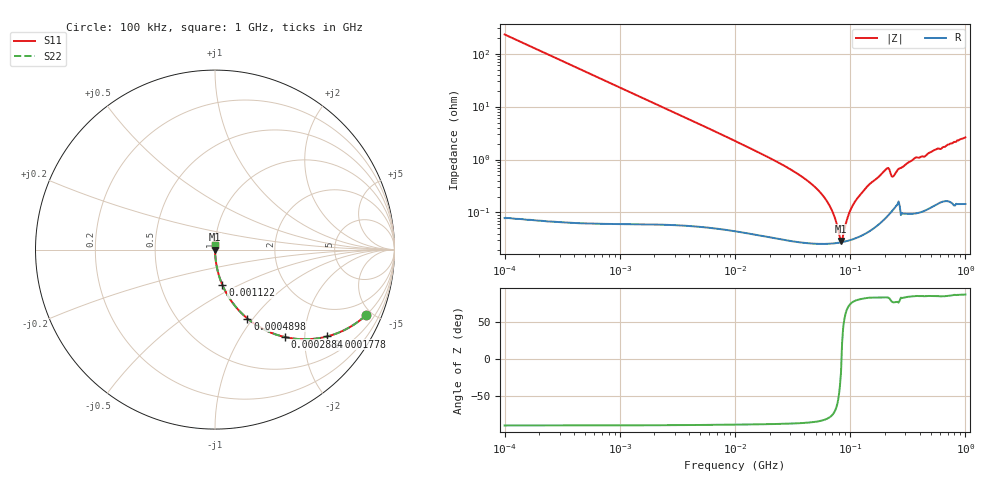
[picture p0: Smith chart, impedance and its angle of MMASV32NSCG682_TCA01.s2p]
! MMASV32NSCG682_TCA01  S-PARAMETER MODEL  ( Standard Model )
! Model Generated by TAIYO YUDEN Corporation (https://www.yuden.co.jp/en/)
! Version 1.0
! TAIYO YUDEN Control No. 250312
! Copyright(c) 2025 TAIYO YUDEN CO.,LTD. All Rights Reserved.
! Product Description (link to TY-COMPAS)
! https://ds.yuden.co.jp/TYCOMPAS/or/detail?pn=MMASV32NSCG682JTCA01&u=M
! Products Name : Multilayer Ceramic Capacitors
! Characteristics :
!  Capacitance : 6800 [pF] , Rated Voltage : 1000 [V] , TCC : CG / C0G
!  Case Size : 3.2 x 2.5 / 0.126 x 0.098 [mm/inch] , Thickness : 1.9 / 0.075 [mm/inch]
!  (Conditions: Temperature = 25 [degC] , DC Bias Voltage = 0 [V])
! External Node Assignments :
!  1  o---| |---o  2
! GND o---------o GND
! Frequency Range : 0.1MHz  -  1000MHz  [ 401 STEP ]
# MHZ S RI R 50
! Freq[MHz].  S11 Real  S11 Imag  S21 Real  S21 Imag  S12 Real  S12 Imag  S22 Real  S22 Imag
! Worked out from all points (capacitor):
!   401 points, 100 kHz to 1 GHz, reference 50 ohm
!   read as one part in series: C = 6.92 nF near 104.7 kHz
!   lowest |Z| = 28.9 mohm at 83.18 MHz (marker M1)
!   series resonance near 84.05 MHz, so ESL is about 520 pH
!   S11 on the Smith chart (normalised r, x): 100 kHz: 1.00, -4.60; 177.8 kHz: 1.00, -2.59; 288.4 kHz: 1.00, -1.60; 489.8 kHz: 1.00, -0.94; 1.122 MHz: 1.00, -0.41; 1 GHz: 1.00, +0.05
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0.1  0.8411 -0.3654  0.1589 0.3654  0.1589 0.3654  0.8411 -0.3654
0.177828  0.6259 -0.4836  0.3741 0.4836  0.3741 0.4836  0.6259 -0.4836
0.288403  0.3889 -0.4871  0.6111 0.4871  0.6111 0.4871  0.3889 -0.4871
0.467735  0.195 -0.3956  0.805 0.3956  0.805 0.3956  0.195 -0.3956
0.489779  0.181 -0.3844  0.819 0.3844  0.819 0.3844  0.181 -0.3844
1.122018  0.0408 -0.1964  0.9592 0.1964  0.9592 0.1964  0.0408 -0.1964
2.187762  0.0115 -0.1037  0.9885 0.1037  0.9885 0.1037  0.0115 -0.1037
10  0.000946 -0.0224  0.9991 0.0224  0.9991 0.0224  0.000946 -0.0224
26.91535  0.000359 -0.00757  0.9996 0.00757  0.9996 0.00757  0.000359 -0.00757
46.77351  0.00027 -0.00336  0.9997 0.00336  0.9997 0.00336  0.00027 -0.00336
66.06934  0.000259 -0.00134  0.9997 0.00134  0.9997 0.00134  0.000259 -0.00134
72.4436  0.000262 -0.000832  0.9997 0.000832  0.9997 0.000832  0.000262 -0.000832
81.28305  0.000271 -0.000211  0.9997 0.000211  0.9997 0.000211  0.000271 -0.000211
83.17638  0.000273 -9.38e-05  0.9997 9.38e-05  0.9997 9.38e-05  0.000273 -9.38e-05
87.09636  0.000279 0.000267  0.9997 -0.000267  0.9997 -0.000267  0.000279 0.000267
100  0.000302 0.00104  0.9997 -0.00104  0.9997 -0.00104  0.000302 0.00104
114.8154  0.000338 0.0018  0.9997 -0.0018  0.9997 -0.0018  0.000338 0.0018
204.1738  0.000835 0.00646  0.9992 -0.00646  0.9992 -0.00646  0.000835 0.00646
218.7762  0.000972 0.00643  0.999 -0.00643  0.999 -0.00643  0.000972 0.00643
239.8833  0.0012 0.00483  0.9988 -0.00483  0.9988 -0.00483  0.0012 0.00483
363.0781  0.00107 0.0106  0.9989 -0.0106  0.9989 -0.0106  0.00107 0.0106
1000  0.00213 0.0261  0.9979 -0.0261  0.9979 -0.0261  0.00213 0.0261
